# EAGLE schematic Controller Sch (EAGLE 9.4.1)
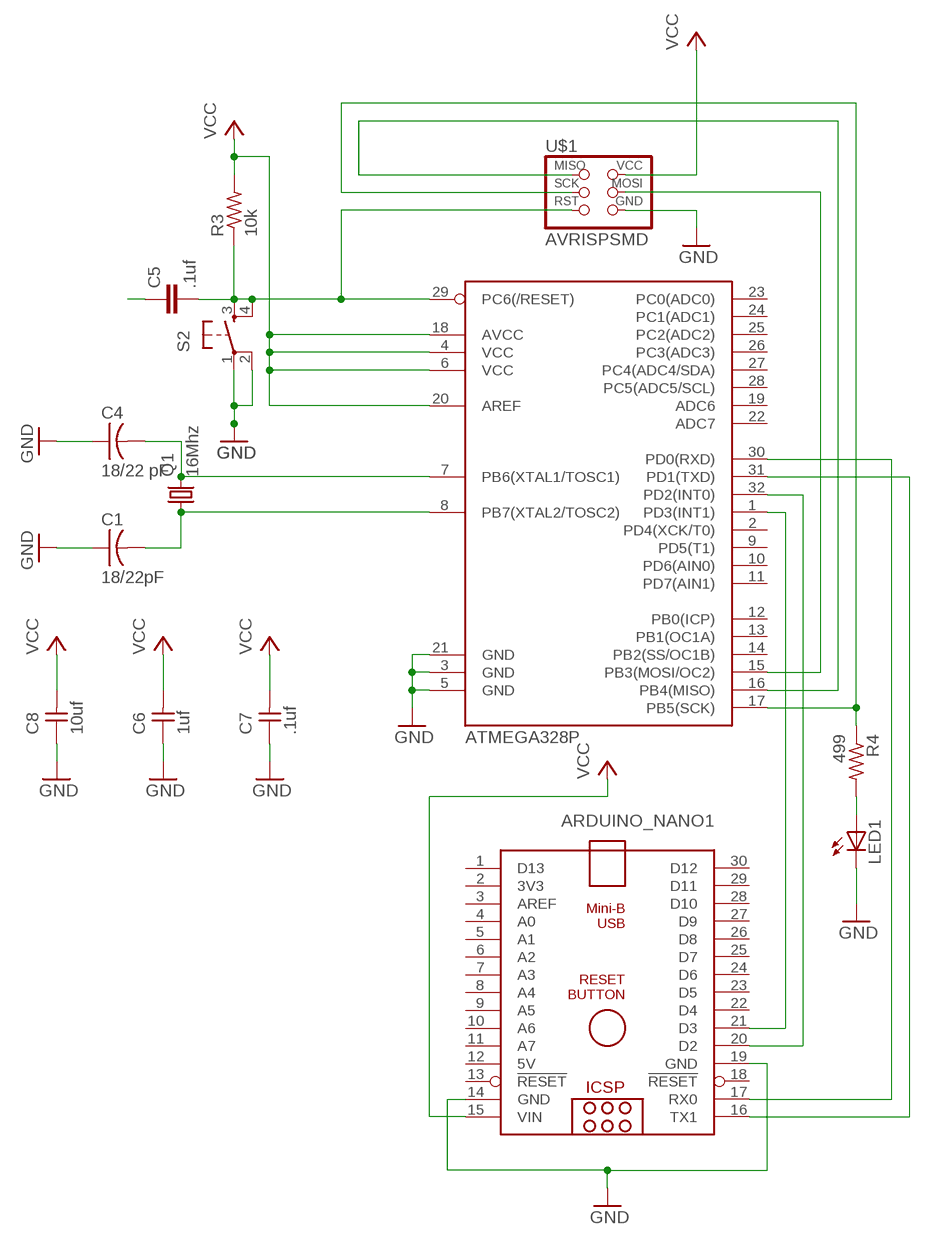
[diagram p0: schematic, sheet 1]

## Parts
ARDUINO_NANO1  ARDUINO_NANO  [ARDUINO_NANO]
ATMEGA328P  ATMEGA88-THIN  [TQFP32-08THIN]
C1  18/22pF  CAP-US1206FAB  [C1206FAB]
C4  18/22 pF  CAP-US1206FAB  [C1206FAB]
C5  .1uf  C-EUC1206  [C1206]
C6  1uf  UNPOLARIZED_CAPACITOR1206  [1206]
C7  .1uf  UNPOLARIZED_CAPACITOR1206  [1206]
C8  10uf  UNPOLARIZED_CAPACITOR1206  [1206]
LED1  LED1206  [1206]
Q1  16Mhz  CSM-7X-DU  [CSM-7X-DU]
R3  10k  RESISTOR1206  [1206]
R4  499  RESISTOR1206  [1206]
S2  6MM_SWITCH6MM_SWITCH  [6MM_SWITCH]
U$1  AVRISPSMD  [2X03SMD]

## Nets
GND: ARDUINO_NANO1.14(GND) ARDUINO_NANO1.19(GND) ATMEGA328P.3(GND) ATMEGA328P.5(GND) ATMEGA328P.21(GND) C1.1 C4.1 C6.1 C7.1 C8.1 LED1.2(C) S2.1(P) S2.2(P1) U$1.6(GND)
N$1: ATMEGA328P.8(PB7(XTAL2/TOSC2)) C1.2 Q1.1
N$2: ATMEGA328P.7(PB6(XTAL1/TOSC1)) C4.2 Q1.2
N$16: ATMEGA328P.15(PB3(MOSI/OC2)) U$1.4(MOSI)
N$19: ATMEGA328P.16(PB4(MISO)) U$1.1(MISO)
N$20: ATMEGA328P.17(PB5(SCK)) R4.1 U$1.3(SCK)
N$21: LED1.1(A) R4.2
N$25: C5.1
N$26: ARDUINO_NANO1.17(RX0) ATMEGA328P.30(PD0(RXD))
N$27: ARDUINO_NANO1.21(D3) ATMEGA328P.1(PD3(INT1))
N$28: ARDUINO_NANO1.20(D2) ATMEGA328P.32(PD2(INT0))
N$29: ARDUINO_NANO1.16(TX1) ATMEGA328P.31(PD1(TXD))
RST1: ATMEGA328P.29(PC6(/RESET)) C5.2 R3.1 S2.3(S) S2.4(S1) U$1.5(RST)
VCC: ARDUINO_NANO1.15(VIN) ATMEGA328P.4(VCC) ATMEGA328P.6(VCC) ATMEGA328P.18(AVCC) ATMEGA328P.20(AREF) C6.2 C7.2 C8.2 R3.2 U$1.2(VCC)
Unconnected: ARDUINO_NANO1.1(D13) ARDUINO_NANO1.2(3V3) ARDUINO_NANO1.3(AREF) ARDUINO_NANO1.4(A0) ARDUINO_NANO1.5(A1) ARDUINO_NANO1.6(A2) ARDUINO_NANO1.7(A3) ARDUINO_NANO1.8(A4) ARDUINO_NANO1.9(A5) ARDUINO_NANO1.10(A6) ARDUINO_NANO1.11(A7) ARDUINO_NANO1.13(!RESET) ARDUINO_NANO1.18(!RESET) ARDUINO_NANO1.22(D4) ARDUINO_NANO1.23(D5) ARDUINO_NANO1.24(D6) ARDUINO_NANO1.25(D7) ARDUINO_NANO1.26(D8) ARDUINO_NANO1.27(D9) ARDUINO_NANO1.28(D10) ARDUINO_NANO1.29(D11) ARDUINO_NANO1.30(D12) ATMEGA328P.2(PD4(XCK/T0)) ATMEGA328P.9(PD5(T1)) ATMEGA328P.10(PD6(AIN0)) ATMEGA328P.11(PD7(AIN1)) ATMEGA328P.12(PB0(ICP)) ATMEGA328P.13(PB1(OC1A)) ATMEGA328P.14(PB2(SS/OC1B)) ATMEGA328P.19(ADC6) ATMEGA328P.22(ADC7) ATMEGA328P.23(PC0(ADC0)) ATMEGA328P.24(PC1(ADC1)) ATMEGA328P.25(PC2(ADC2)) ATMEGA328P.26(PC3(ADC3)) ATMEGA328P.27(PC4(ADC4/SDA)) ATMEGA328P.28(PC5(ADC5/SCL))

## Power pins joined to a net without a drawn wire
5V: ARDUINO_NANO1.12(5V)

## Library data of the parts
ARDUINO_NANO1 = ArduinoNanoV30:ARDUINO_NANO: Arduino Nano V3.0 Overview: The Arduino Nano is a small, complete, and breadboard-friendly board based on the ATmega328 (Arduino Nano 3.x) or ATmega168 (Arduino Nano 2.x). It has more or less the same functionality of the Arduino Duemilanove, but in a different package. It lacks only a DC power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
ATMEGA328P = 1_fab:ATMEGA88-THIN
C1 C4 = 1_fab:CAP-US
C5 = rcl:C-EU: CAPACITOR, European symbol
C6-C8 = ng:UNPOLARIZED_CAPACITOR: unpolarized_capacitor
LED1 = ng:LED
Q1 = crystal:CSM-7X-DU: SMD CRYSTAL; OC_FARNELL: unknown; OC_NEWARK: unknown
R3 R4 = ng:RESISTOR
S2 = ng:6MM_SWITCH: OMRON SWITCH
U$1 = fab:AVRISP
